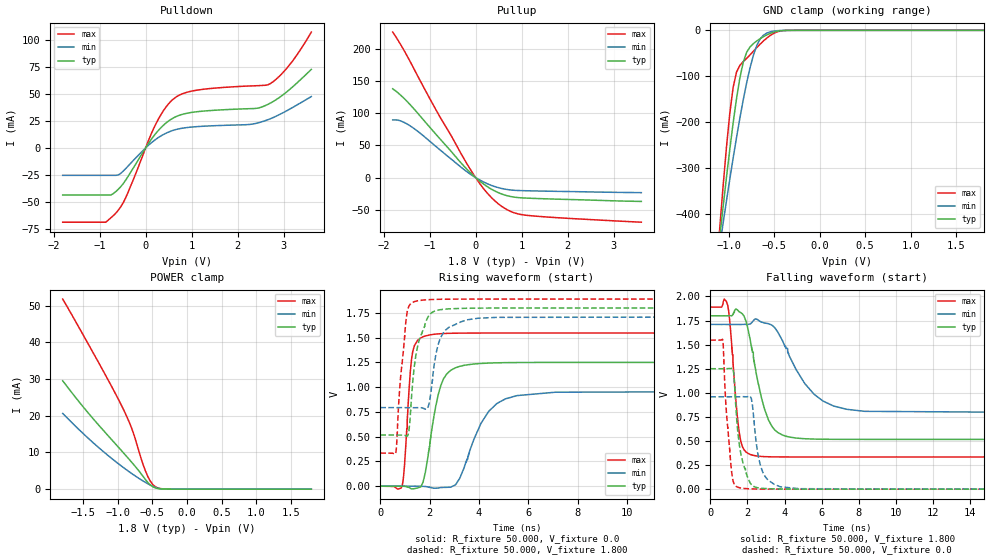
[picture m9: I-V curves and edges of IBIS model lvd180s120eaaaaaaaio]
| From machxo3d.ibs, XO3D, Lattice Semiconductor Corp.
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|   Model lvd180s120eaaaaaaaio
[Model] lvd180s120eaaaaaaaio
Model_type I/O
Polarity   Non-Inverting
Enable   Active-Low
Vinl =  0.630V
Vinh =  1.170V
Vmeas =  0.900V
Cref =  0.0F
Rref =  1.000M
Vref =  0.0V
C_comp   4.200pF   3.800pF   7.500pF
[Temperature Range]   25.000   0.105k   -40.000
[Voltage Range]   1.800V   1.710V   1.890V
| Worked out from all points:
|   slope of the pulldown table from 0 to 0.27 V, typ, clamps not added: 17 ohm
|   slope of the pullup table from 0 to 0.27 V, typ, clamps not added: 18.2 ohm
|   GND clamp passes 1 mA (typ) near -0.43 V on its own axis
|   POWER clamp passes 1 mA (typ) near -0.52 V on its own axis
|   rising waveform, R_fixture 50.000, V_fixture 0.0: 20-80 % time 534ps typ, 1.04ns min, 241ps max; typ from 0 V to 1.25 V
|   rising waveform, R_fixture 50.000, V_fixture 1.800: 20-80 % time 458ps typ, 434ps min, 300ps max; typ from 0.517 V to 1.8 V
|   falling waveform, R_fixture 50.000, V_fixture 1.800: 20-80 % time 875ps typ, 1.73ns min, 401ps max; typ from 1.8 V to 0.517 V
|   falling waveform, R_fixture 50.000, V_fixture 0.0: 20-80 % time 463ps typ, 474ps min, 336ps max; typ from 1.25 V to 0 V
[Pulldown]
|Voltage   I(typ)   I(min)   I(max)
-1.8V     -43.55mA   -25.31mA   -68.69mA
-865mV    -43.55mA   -25.31mA   -68.69mA
-645mV    -40.3mA    -25.31mA   -60.23mA
-425mV    -29.3mA    -18.76mA   -45.41mA
235mV     14.17mA    8.428mA    23.27mA
455mV     23.55mA    13.92mA    38.6mA
620mV     28.2mA     16.61mA    45.89mA
1.115V    33.56mA    19.78mA    53.54mA
2.38V     36.6mA     22.62mA    57.6mA
2.71V     41.55mA    27.09mA    59.61mA
3.15V     54.96mA    36.45mA    78.16mA
3.6V      72.76mA    47.57mA    107.3mA
[Pullup]
|Voltage   I(typ)   I(min)   I(max)
-1.8V     137.8mA    89.5mA     225.8mA
-1.625V   127.7mA    87.86mA    206.1mA
-1.35V    107.5mA    76.77mA    170.4mA
-800mV    62.24mA    44.62mA    97.43mA
-140mV    9.467mA    6.582mA    15.76mA
25mV      -1.58mA    -1.08mA    -2.674mA
190mV     -10.93mA   -7.424mA   -18.66mA
355mV     -18.44mA   -12.42mA   -31.8mA
520mV     -24.17mA   -16.11mA   -42.18mA
795mV     -29.88mA   -19.49mA   -53.5mA
1.07V     -31.75mA   -20.4mA    -58.22mA
3.6V      -37.02mA   -23.41mA   -69.25mA
[GND_clamp]
|Voltage   I(typ)   I(min)   I(max)
-1.8V     -1.831A    -1.488A    -2.421A
-1.097V   -451mA     -469.7mA   -431.6mA
-1.06V    -384.8mA   -420mA     -340.3mA
-986mV    -258.9mA   -323.6mA   -180.7mA
-949mV    -200.9mA   -277.4mA   -123.7mA
-912mV    -148.2mA   -232.8mA   -90.76mA
-838mV    -69.05mA   -150.6mA   -67.91mA
-801mV    -47.74mA   -114.1mA   -60.88mA
-690mV    -23.16mA   -33.02mA   -37.51mA
-579mV    -9.79mA    -5.846mA   -16.62mA
-357mV    -148.7uA   -66.38uA   -242.3uA
1.8V      0A         0A         0A
[POWER_clamp]
|Voltage   I(typ)   I(min)   I(max)
-1.8V     29.51mA    20.63mA    51.76mA
-1.345V   18.87mA    12.41mA    36.66mA
-938mV    10.26mA    6.136mA    22.4mA
-864mV    8.689mA    5.106mA    19.43mA
-790mV    7.087mA    4.117mA    16.01mA
-679mV    4.54mA     2.724mA    9.207mA
-605mV    2.701mA    1.871mA    5.102mA
-531mV    1.131mA    1.1mA      2.169mA
-457mV    338.1uA    470.7uA    629.2uA
-383mV    89.2uA     117.2uA    163.1uA
-272mV    9.185uA    9.485uA    15.7uA
1.8V      0A         0A         4.279nA
[Ramp]
| variable   typ   min   max
dV/dt_r   0.750/0.533n   0.575/1.035n   0.928/0.239n
dV/dt_f   0.770/0.868n   0.550/1.738n   0.933/0.399n
R_load = 50.000
[Rising Waveform]
R_fixture= 50.000
V_fixture= 0.0
V_fixture_min= 0.0
V_fixture_max= 0.0
|time   V(typ)   V(min)   V(max)
0s        5.055nV    47.21nV    2.607nV
885ps     -658.1uV   -14.04uV   1.824mV
984ps     -1.816mV   -136.3uV   215.5mV
1.27ns    -27.83mV   -223.1uV   1.287V
1.828ns   139.9mV    -3.466mV   1.517V
2.45ns    1.014V     -14.09mV   1.54V
3.223ns   1.211V     80.22mV    1.546V
4.398ns   1.243V     756.4mV    1.547V
5.544ns   1.249V     914.9mV    1.547V
20ns      1.25V      958.6mV    1.547V
[Rising Waveform]
R_fixture= 50.000
V_fixture= 1.800
V_fixture_min= 1.710
V_fixture_max= 1.890
|time   V(typ)   V(min)   V(max)
0s        516.8mV    793.5mV    334.2mV
633ps     516.2mV    793.5mV    343.7mV
815ps     516.1mV    793.5mV    1.076V
1.054ns   506.5mV    792.9mV    1.701V
1.164ns   565.5mV    792.7mV    1.819V
1.437ns   1.312V     792.7mV    1.868V
2.056ns   1.746V     952.8mV    1.885V
2.509ns   1.785V     1.531V     1.888V
3.539ns   1.797V     1.681V     1.89V
20ns      1.8V       1.71V      1.89V
[Falling Waveform]
R_fixture= 50.000
V_fixture= 1.800
V_fixture_min= 1.710
V_fixture_max= 1.890
|time   V(typ)   V(min)   V(max)
0s        1.8V       1.71V      1.89V
937ps     1.8V       1.71V      1.912V
1.553ns   1.842V     1.71V      595.8mV
2.154ns   1.547V     1.715V     360.5mV
2.747ns   955.7mV    1.735V     339.7mV
3.136ns   718.3mV    1.718V     336.3mV
4.073ns   549.6mV    1.461V     334.4mV
5.587ns   519.9mV    986.3mV    334.2mV
7.366ns   517mV      828.5mV    334.2mV
20ns      516.8mV    793.4mV    334.2mV
[Falling Waveform]
R_fixture= 50.000
V_fixture= 0.0
V_fixture_min= 0.0
V_fixture_max= 0.0
|time   V(typ)   V(min)   V(max)
0s        1.25V      958.6mV    1.547V
675ps     1.25V      958.6mV    1.546V
834ps     1.251V     958.5mV    900.1mV
1.138ns   1.254V     958.6mV    198.3mV
1.264ns   1.202V     958.6mV    64.27mV
1.488ns   583.3mV    959mV      19.8mV
2.21ns    48.34mV    942.7mV    3.061mV
2.722ns   10.18mV    232.2mV    753.3uV
3.768ns   1.969mV    25.1mV     117uV
20ns      10.61nV    109.6nV    -15.16nV
